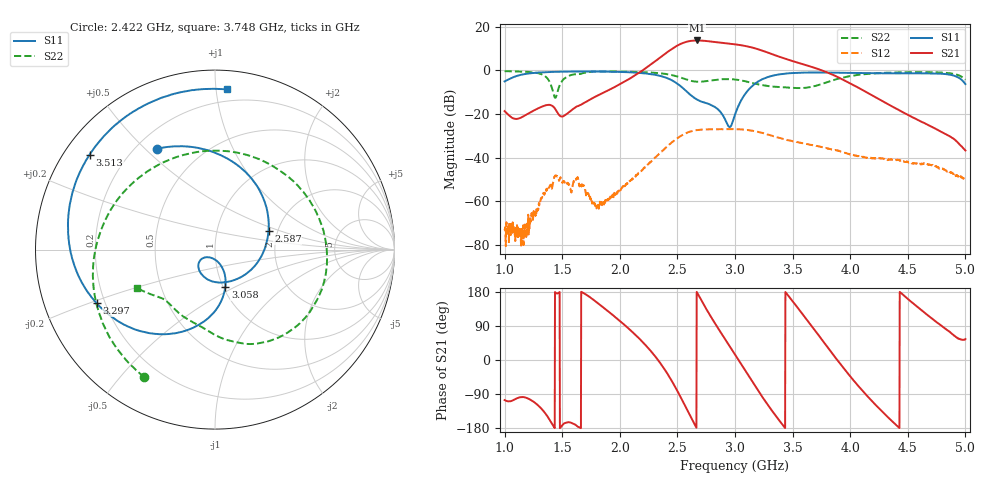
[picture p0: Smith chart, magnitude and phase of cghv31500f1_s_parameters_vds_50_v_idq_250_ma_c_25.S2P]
!Keysight Technologies,E5071C,MY46632031,B.14.03
!Date: Fri Jul 09 16:08:11 2021
!Data & Calibration Information:
!Freq	S11:SOLT2(ON)	S21:SOLT2(ON)	S12:SOLT2(ON)	S22:SOLT2(ON)
!PortZ  Port1:50+j0  Port2:50+j0
!Above PortZ is port z conversion or system Z0 setting when saving the data.
!When reading, reference impedance value at option line is always used.
# Hz S dB R 50
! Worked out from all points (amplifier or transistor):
!   1601 points, 1 GHz to 5 GHz, reference 50 ohm
!   highest |S21| = 13.8 dB at 2.67 GHz (marker M1)
!   |S21| within 3 dB of that: 2.478 GHz to 3.13 GHz (652.1 MHz wide, 23.3 % of centre)
!   unconditionally stable (mu >= 1): start of sweep to end of sweep
!   at 1.665 GHz: K = 36.65, MAG = -0.2 dB, |S12| = -52.5 dB
!   at 3 GHz: K = 1.77, MAG = 14.4 dB, |S12| = -27.0 dB
!   at 5 GHz: K = 5331.27, MAG = -33.5 dB, |S12| = -50.3 dB
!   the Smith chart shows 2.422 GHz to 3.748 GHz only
!   S11 on the Smith chart (normalised r, x): 2.422 GHz: 0.28, +0.54; 2.587 GHz: 1.79, +0.42; 3.058 GHz: 1.02, -0.45; 3.297 GHz: 0.17, -0.21; 3.513 GHz: 0.07, +0.33; 3.748 GHz: 0.12, +1.07
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1e9  -5.01 154.0  -18.64 -105.8  -73.31 134.6  -0.33 122.7
1.315e9  -0.89 75.5  -16.78 -126.9  -58.64 -132.0  -1.61 61.7
1.6675e9  -0.47 -15.2  -15.57 179.6  -53.20 -162.9  -1.41 54.9
2.065e9  -0.79 -115.2  -4.41 86.1  -51.69 1.3  -0.57 -21.9
2.335e9  -2.30 158.8  5.31 -1.5  -38.57 -85.6  -1.20 -87.6
2.4225e9  -3.76 120.1  8.79 -40.6  -34.29 -124.5  -1.81 -119.1
2.52e9  -6.87 65.3  11.97 -93.3  -30.33 -177.3  -3.11 -166.5
2.5875e9  -10.00 19.4  13.27 -133.3  -28.46 143.3  -4.29 152.8
2.67e9  -13.33 -42.0  13.76 178.4  -27.35 94.8  -5.16 98.6
2.75e9  -14.96 -93.3  13.51 135.0  -27.04 51.9  -4.91 51.8
2.8225e9  -16.66 -126.3  13.07 98.5  -26.98 15.4  -4.37 17.3
2.9e9  -21.06 -145.0  12.59 61.5  -26.94 -21.5  -3.99 -12.9
3e9  -20.24 -69.2  11.96 14.4  -26.96 -68.4  -4.15 -45.3
3.0575e9  -13.33 -74.5  11.53 -12.9  -27.04 -95.7  -4.62 -61.0
3.1725e9  -6.12 -112.0  10.18 -67.7  -27.84 -149.8  -6.03 -84.5
3.2975e9  -2.82 -155.5  7.95 -123.9  -29.58 153.9  -7.23 -101.0
3.5125e9  -1.15 142.8  4.09 150.2  -32.53 69.3  -8.02 -127.0
3.6675e9  -0.94 104.6  1.61 89.0  -34.22 9.6  -7.47 -142.8
3.7475e9  -0.96 85.6  0.17 56.5  -35.03 -21.2  -6.30 -153.9
4.335e9  -1.31 -65.2  -15.66 -153.2  -40.94 171.0  -1.03 63.6
4.7e9  -1.35 -165.2  -25.62 111.6  -43.32 89.1  -0.81 -0.5
5e9  -6.24 120.2  -36.70 55.0  -50.30 32.8  -4.26 -50.0
